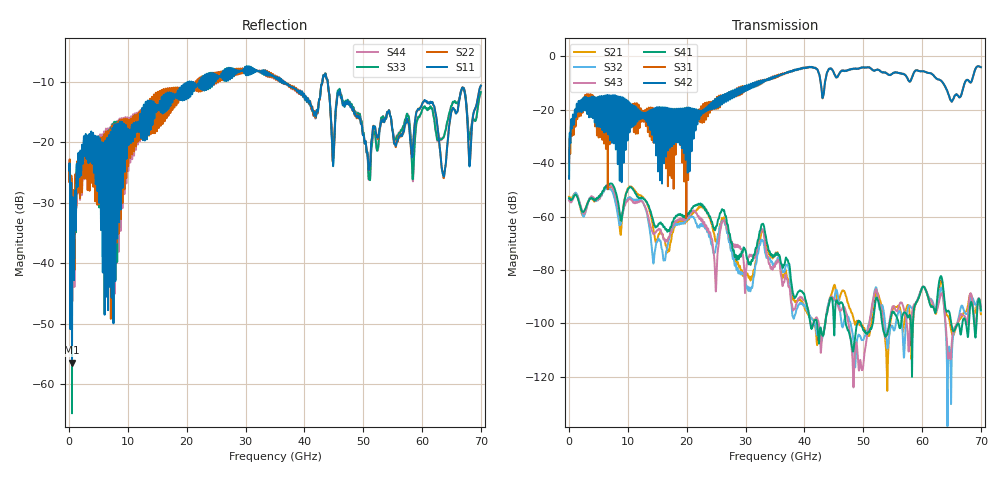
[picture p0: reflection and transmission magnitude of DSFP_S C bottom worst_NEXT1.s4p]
! AWR Design Environment (8415) Wed Jan 09 13:29:16 2019
! Document = 'DSFP_S'
! nPorts: 4, nXvals: 7001
# HZ S DB R 50
!Freq DBS11 AngS11 DBS12 AngS12 DBS13 AngS13 DBS14 AngS14
!	DBS21 AngS21 DBS22 AngS22 DBS23 AngS23 DBS24 AngS24
!	DBS31 AngS31 DBS32 AngS32 DBS33 AngS33 DBS34 AngS34
!	DBS41 AngS41 DBS42 AngS42 DBS43 AngS43 DBS44 AngS44
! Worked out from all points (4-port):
!   7000 points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, 10 MHz to 70 GHz, reference 50 ohm
!   strongest paths, dB at 10 MHz, 17.51 GHz, 35.01 GHz, 52.51 GHz, 70 GHz:
!     S42: -45.8, -29.4, -7.6, -5.0, -4.0
!     S31: -39.6, -26.7, -7.3, -4.9, -4.0
!     S41: -53.1, -62.2, -74.4, -91.4, -94.9
!     S43: -54.0, -63.8, -78.3, -89.8, -94.0
!     S32: -53.5, -64.2, -78.1, -90.5, -95.4
!     S21: -52.6, -66.2, -74.3, -88.8, -96.5
!   lowest |S11| = -56.5 dB at 500 MHz (marker M1), VSWR 1.00, Z = 50 + j0.146 ohm
!   |S11| at or under -10 dB: start of sweep to 20.42 GHz; 36.43 GHz to 43.08 GHz (6.652 GHz wide, 16.7 % of centre); 43.95 GHz to end of sweep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
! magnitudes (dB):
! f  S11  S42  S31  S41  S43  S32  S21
! 10 MHz  -24.7  -45.8  -39.6  -53.1  -54.0  -53.5  -52.6
! 500 MHz  -56.5  -26.6  -29.8  -53.5  -54.2  -53.4  -52.8
! 12.25 GHz  -19.2  -23.3  -21.8  -52.9  -54.1  -53.7  -52.1
! 16.2 GHz  -14.7  -23.5  -27.4  -63.8  -68.3  -75.9  -68.3
! 26.26 GHz  -8.3  -15.6  -16.5  -57.6  -61.4  -61.5  -60.4
! 29.47 GHz  -8.3  -11.8  -11.1  -73.4  -73.6  -81.6  -81.8
! 70 GHz  -10.7  -4.0  -4.0  -94.9  -94.0  -95.4  -96.5
